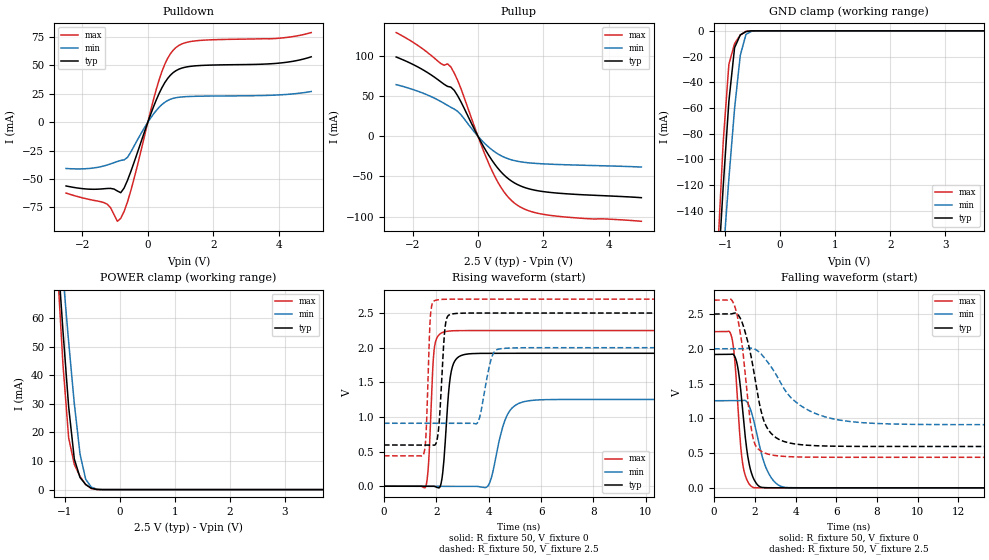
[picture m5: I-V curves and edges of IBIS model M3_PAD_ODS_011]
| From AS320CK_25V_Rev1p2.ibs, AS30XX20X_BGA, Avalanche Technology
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[Model] M3_PAD_ODS_011
Model_type I/O
Enable   Active-High
Vinl  =  0.7
Vinh  =  1.8
Vmeas =  1.25
Cref  =  30e-12
| Capacitance  typ   min   max
C_comp   1.568193e-12   1.472592e-12   1.715469e-12
| Variables   typ   min   max
[GND Clamp Reference]   0   0   0
[POWER Clamp Reference]   2.5   2   2.7
[Pulldown Reference]   0   0   0
[Pullup Reference]   2.5   2   2.7
[Temperature Range]   25   125   -40
[Voltage Range]   2.5   2   2.7
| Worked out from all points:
|   slope of the pulldown table from 0 to 0.375 V, typ, clamps not added: 13.9 ohm
|   slope of the pullup table from 0 to 0.375 V, typ, clamps not added: 14.1 ohm
|   GND clamp passes 1 mA (typ) near -0.64 V on its own axis
|   POWER clamp passes 1 mA (typ) near -0.56 V on its own axis
|   falling waveform, R_fixture 50, V_fixture 0: 20-80 % time 436ps typ, 691ps min, 330ps max; typ from 1.92 V to 0 V
|   falling waveform, R_fixture 50, V_fixture 2.5: 20-80 % time 793ps typ, 1.86ns min, 532ps max; typ from 2.5 V to 0.595 V
|   rising waveform, R_fixture 50, V_fixture 0: 20-80 % time 226ps typ, 493ps min, 156ps max; typ from 0 V to 1.92 V
|   rising waveform, R_fixture 50, V_fixture 2.5: 20-80 % time 174ps typ, 327ps min, 120ps max; typ from 0.595 V to 2.5 V
[GND Clamp]
| Voltage   I(typ)   I(min)   I(max)
-2.5V     -1.297A    -1.146A    -1.538A
-1.138V   -195.9mA   -238.3mA   -175.2mA
-1.034V   -121.2mA   -175.1mA   -86.57mA
-931mV    -54.79mA   -114.9mA   -26.01mA
-827.6mV  -13.15mA   -60.41mA   -9.967mA
-724.1mV  -3.205mA   -19.15mA   -3.28mA
-620.7mV  -615.3uA   -2.798mA   -407.6uA
-517.2mV  -34.39uA   -319.4uA   -6.513uA
-413.8mV  -821.3nA   -24.43uA   -50.96nA
5V        0A         0A         0A
[POWER Clamp]
| Voltage   I(typ)   I(min)   I(max)
-2.5V     511mA      454.9mA    606.6mA
-1.138V   84.76mA    99.9mA     78.64mA
-1.034V   55.67mA    75.27mA    43.94mA
-931mV    29.07mA    51.7mA     18.16mA
-827.6mV  10.68mA    30.08mA    8.788mA
-724.1mV  4.238mA    12.45mA    4.618mA
-620.7mV  1.771mA    3.587mA    1.776mA
-517.2mV  465uA      837.9uA    329.7uA
-413.8mV  47.65uA    120.2uA    11.19uA
-310.3mV  1.515uA    11.72uA    116.8nA
5V        0A         0A         0A
[Pulldown]
| Voltage   I(typ)   I(min)   I(max)
-2.5V     -56.05mA   -40.67mA   -62.34mA
-1.345V   -58.52mA   -38.46mA   -70.65mA
-1.138V   -58.21mA   -36.64mA   -75.26mA
-931mV    -60.47mA   -34.5mA    -87.15mA
-827.6mV  -61.98mA   -33.61mA   -84.55mA
-517.2mV  -43.17mA   -26.04mA   -59.93mA
344.8mV   25.28mA    13.14mA    37.23mA
603.4mV   38.43mA    19.08mA    56.07mA
948.3mV   46.68mA    21.99mA    67.55mA
1.638V    49.99mA    22.96mA    72.11mA
3.99V     51.98mA    24.03mA    73.9mA
5V        57.62mA    27.08mA    78.94mA
[Pullup]
| Voltage   I(typ)   I(min)   I(max)
-2.5V     98.57mA    64.21mA    129mA
-1.759V   84.42mA    54.83mA    110.7mA
-1.138V   67.76mA    43.28mA    90.53mA
-827.6mV  61.06mA    35.97mA    86.19mA
-517.2mV  42.68mA    26.63mA    59.02mA
86.21mV   -6.592mA   -3.867mA   -9.337mA
431mV     -29.98mA   -16.93mA   -42.94mA
775.9mV   -47.31mA   -25.59mA   -67.97mA
1.121V    -58.14mA   -30.35mA   -83.25mA
1.552V    -65.3mA    -33.06mA   -92.67mA
2.155V    -69.64mA   -34.65mA   -98.12mA
5V        -76.42mA   -38.32mA   -105.8mA
[Ramp]
dV/dt_r   1.15105/0.226491n  0.751697/0.493289n  1.34788/0.15619n
dV/dt_f   1.14297/0.792607n  0.654869/1.86468n  1.35646/0.5318n
R_load = 50
[Falling Waveform]
R_fixture = 50
V_fixture = 0
V_fixture_min = 0
V_fixture_max = 0
| Time   V(typ)   V(min)   V(max)
0s        1.918V     1.253V     2.246V
852.3ps   1.922V     1.253V     2.184V
996.5ps   1.9V       1.253V     1.903V
1.131ns   1.783V     1.253V     1.364V
1.383ns   1.185V     1.256V     390.4mV
1.626ns   508.9mV    1.231V     106.5mV
1.913ns   151.4mV    1.008V     6.78mV
2.595ns   2.191mV    260mV      769.8uV
3.446ns   549uV      8.745mV    735.8uV
21.88ns   354.9nV    2.207uV    -559.4nV
[Falling Waveform]
R_fixture = 50
V_fixture = 2.5
V_fixture_min = 2
V_fixture_max = 2.7
| Time   V(typ)   V(min)   V(max)
0s        2.5V       2V         2.7V
810.5ps   2.501V     2V         2.714V
1.055ns   2.513V     2.001V     2.575V
1.363ns   2.39V      2.001V     2.086V
1.888ns   1.781V     2.007V     752.7mV
2.491ns   930.4mV    1.863V     500.5mV
3.039ns   722.7mV    1.633V     463.4mV
3.933ns   633.1mV    1.255V     445.9mV
6.147ns   598.2mV    975.7mV    439.5mV
21.88ns   595.1mV    908.6mV    439.2mV
[Rising Waveform]
R_fixture = 50
V_fixture = 0
V_fixture_min = 0
V_fixture_max = 0
| Time   V(typ)   V(min)   V(max)
0s        1.888nV    39.39nV    1.619nV
1.597ns   793.7uV    -373uV     -4.215mV
1.918ns   -1.207mV   -447.9uV   1.976V
2.274ns   304.6mV    -531uV     2.225V
2.564ns   1.645V     -598.7uV   2.242V
3.118ns   1.904V     -728.1uV   2.246V
3.983ns   1.918V     10.33mV    2.246V
4.678ns   1.918V     1.003V     2.246V
5.443ns   1.918V     1.228V     2.246V
21.88ns   1.918V     1.253V     2.246V
[Rising Waveform]
R_fixture = 50
V_fixture = 2.5
V_fixture_min = 2
V_fixture_max = 2.7
| Time   V(typ)   V(min)   V(max)
0s        595.1mV    908.6mV    439.2mV
1.523ns   594.7mV    909mV      472.8mV
1.612ns   594.7mV    909mV      790.9mV
1.773ns   594.7mV    909mV      2.451V
1.993ns   622.1mV    909.1mV    2.686V
2.334ns   2.295V     909.2mV    2.698V
2.554ns   2.481V     909.2mV    2.699V
3.588ns   2.499V     923.9mV    2.7V
4.446ns   2.499V     1.984V     2.7V
21.88ns   2.5V       2V         2.7V
